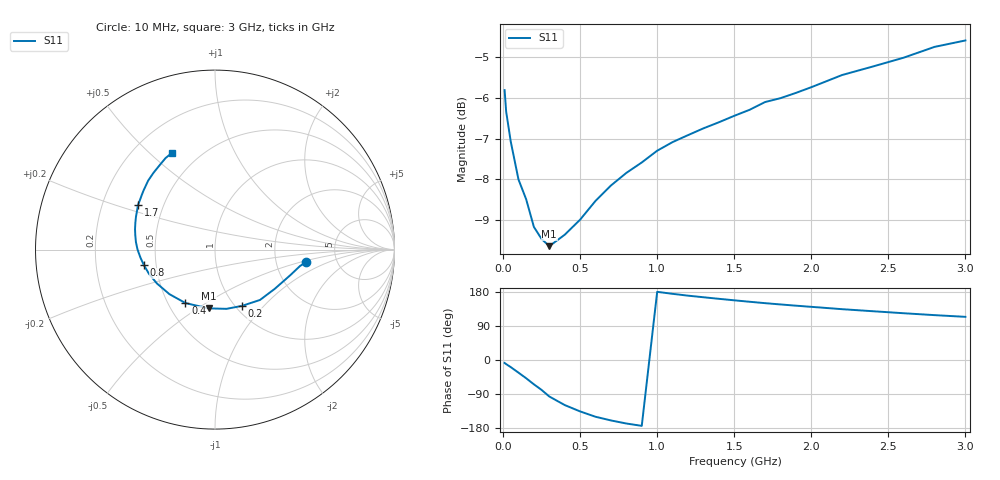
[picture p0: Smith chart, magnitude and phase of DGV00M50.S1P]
! SIEMENS Small Signal Semiconductors
! BAV70
! Silicon Switching Diode in SOT23
! IF = 0.5 mA
! S-Parameters:  May  1995
# GHz  S  MA  R  50
!  f  S11
! GHz  MAG  ANG
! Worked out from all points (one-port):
!   30 points, 10 MHz to 3 GHz, reference 50 ohm
!   lowest |S11| = -9.6 dB at 300 MHz (marker M1), VSWR 1.98, Z = 37.7 - j27.7 ohm
!   |S11| at or under -10 dB: nowhere
!   S11 on the Smith chart (normalised r, x): 10 MHz: 2.98, -0.56; 200 MHz: 1.07, -0.77; 400 MHz: 0.61, -0.41; 800 MHz: 0.43, -0.09; 1.7 GHz: 0.36, +0.24; 3 GHz: 0.36, +0.59
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0.01  0.5127 -7.8
0.02  0.4825 -10.9
0.05  0.4429 -18.8
0.1  0.398 -33.4
0.15  0.3762 -48.2
0.2  0.3479 -64.2
0.25  0.3362 -79.0
0.3  0.3295 -96.3
0.4  0.3403 -118.9
0.5  0.3552 -135.7
0.6  0.3746 -149.8
0.7  0.3913 -159.5
0.8  0.4055 -167.6
0.9  0.4177 -173.8
1  0.4318 179.9
1.1  0.4425 174.6
1.2  0.4513 169.8
1.3  0.46 165.6
1.4  0.468 161.5
1.6  0.4849 153.7
1.7  0.4956 150.0
1.9  0.5086 143.4
2  0.5169 140.3
2.2  0.5351 134.1
2.4  0.5482 128.7
2.6  0.5621 123.4
2.8  0.5795 118.4
3  0.5901 113.9
